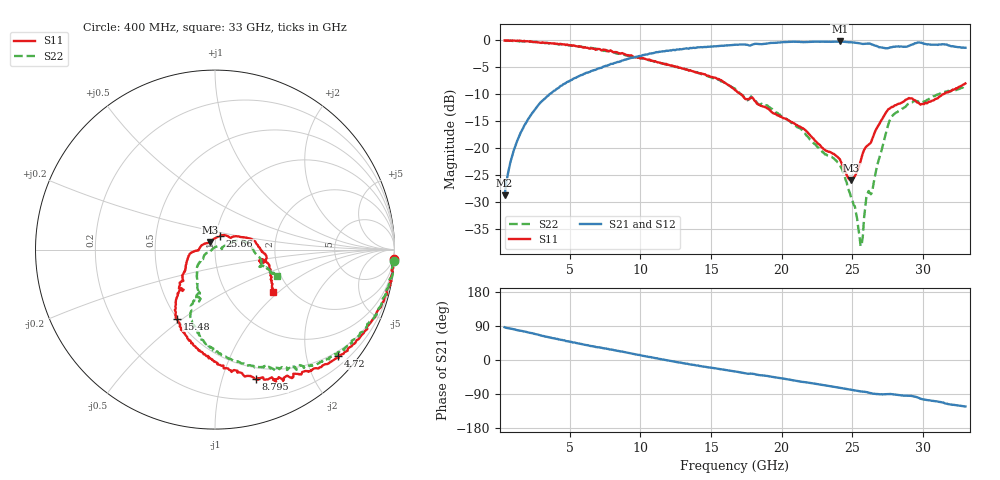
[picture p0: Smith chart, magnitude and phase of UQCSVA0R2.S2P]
!  Part Number  UQCSVA0R2  Mounting Orientation: Horizontal
!  Description: Ultra Low ESR Microwave capacitors
!  Application: Coupling, Bypass, Tuning, DC Block
!  Filters, Matching
# GHZ S DB R 50
! Freq  |S11|  S11 Ph  |S21|  S21 Ph  |S12|  S12 Ph  |S22|  S22 Ph
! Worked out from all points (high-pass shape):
!   401 points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, 400 MHz to 33 GHz, reference 50 ohm
!   highest |S21| = -0.19 dB at 24.12 GHz (marker M1); lowest = -28.7 dB at 400 MHz (marker M2)
!   |S21| within 3 dB of the highest: 9.488 GHz to end of sweep
!   lowest |S11| = -25.9 dB at 24.93 GHz (marker M3), VSWR 1.11, Z = 47.1 + j3.99 ohm
!   |S11| at or under -10 dB: 17.14 GHz to 31.39 GHz (14.25 GHz wide, 58.7 % of centre)
!   |S22| runs from -38.2 to 0.0 dB; largest |S21 - S12| = 0.016
!   S11 on the Smith chart (normalised r, x): 400 MHz: 1, -36; 4.72 GHz: 0.39, -2.64; 8.795 GHz: 0.38, -1.29; 15.48 GHz: 0.50, -0.48; 25.66 GHz: 1.05, +0.16; 33 GHz: 1.63, -0.91
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0.4  -0.01 -3.1  -28.74 86.4  -28.65 86.2  -0.01 -3.5
1.052  -0.02 -7.8  -20.38 81.0  -20.33 79.7  -0.05 -10.4
1.867  -0.16 -15.2  -15.50 74.8  -15.52 73.4  -0.23 -16.3
3.008  -0.45 -27.3  -11.35 64.0  -11.35 63.5  -0.37 -24.2
4.72  -0.84 -40.8  -7.94 50.2  -7.93 50.5  -0.85 -37.4
5.861  -1.23 -49.6  -6.42 42.1  -6.39 42.3  -1.19 -44.6
8.795  -2.42 -72.7  -3.70 21.6  -3.74 21.2  -2.48 -63.5
11.321  -4.09 -90.4  -2.12 3.2  -2.07 3.5  -4.06 -80.7
15.478  -7.17 -118.8  -1.06 -23.0  -1.08 -22.9  -7.23 -106.2
16.7  -9.23 -128.1  -0.82 -30.3  -0.79 -30.0  -8.94 -112.5
22.161  -18.03 -174.0  -0.22 -61.3  -0.19 -61.5  -18.78 -139.7
24.117  -22.05 162.6  -0.19 -73.3  -0.19 -73.5  -23.12 -150.2
24.932  -25.89 123.7  -0.34 -78.8  -0.32 -79.0  -29.29 -155.4
25.502  -23.17 81.7  -0.53 -82.5  -0.50 -82.2  -36.17 169.4
25.665  -21.62 69.3  -0.60 -83.2  -0.59 -83.3  -37.95 103.6
26.073  -19.52 41.5  -0.58 -85.2  -0.55 -85.3  -28.50 14.4
26.399  -18.35 36.2  -0.76 -88.5  -0.75 -88.3  -28.13 13.8
27.621  -12.69 8.7  -1.35 -89.9  -1.37 -90.0  -15.00 14.1
29.007  -10.69 -9.1  -1.00 -94.0  -1.01 -93.9  -11.73 -11.4
29.659  -11.57 -16.3  -0.36 -99.4  -0.38 -99.4  -11.34 -20.0
31.126  -10.51 -14.0  -0.76 -110.4  -0.76 -110.3  -9.95 -20.4
33  -7.99 -36.1  -1.36 -122.6  -1.37 -122.8  -8.48 -22.6
